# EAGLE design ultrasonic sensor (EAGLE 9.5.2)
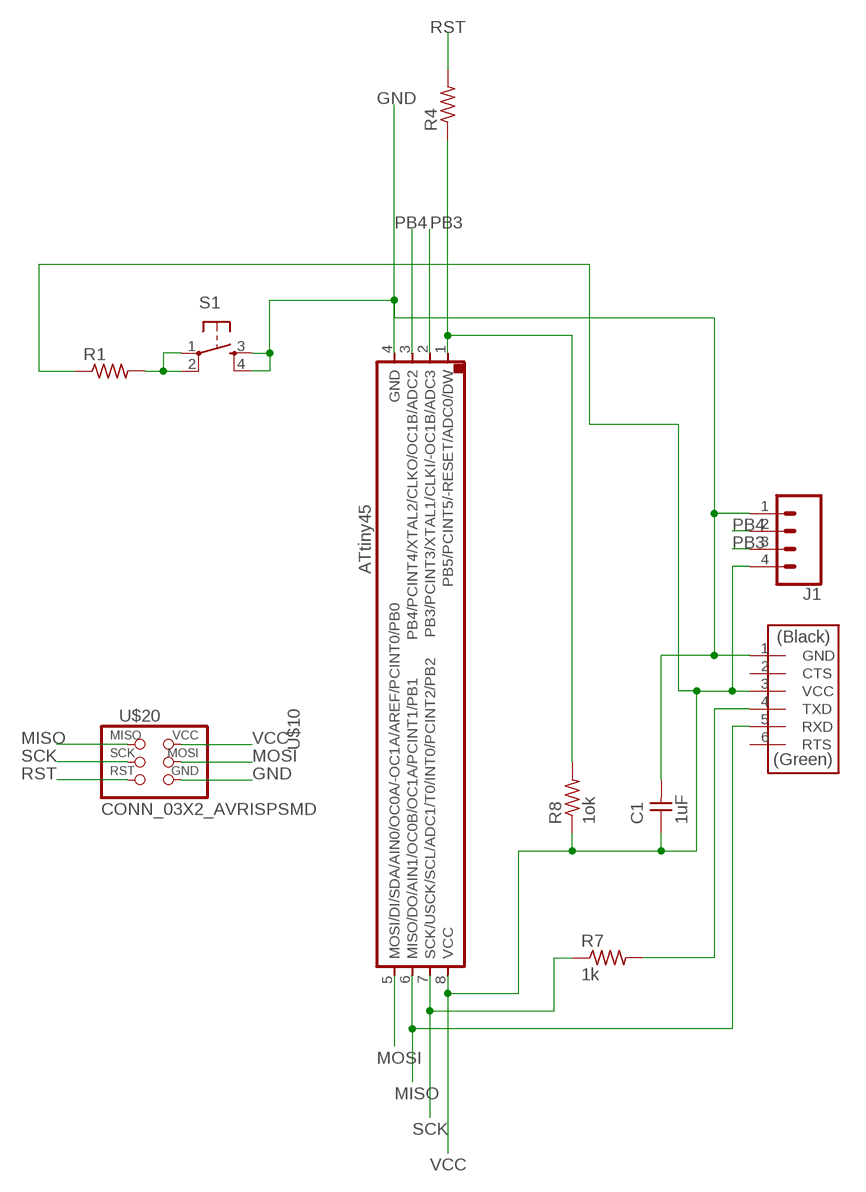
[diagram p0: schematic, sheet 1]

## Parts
C1  1uF  CAP_UNPOLARIZED  [C1206]
J1  CONN_04SMD_RA_FEMALE  [1X04_SMD_RA_FEMALE]
R1  R1206  [R1206]
R4  R1206  [R1206]
R7  1k  R1206  [R1206]
R8  1ok  R1206  [R1206]
S1  SW_SWITCH_TACTILE_6MM6MM_SWITCH  [6MM_SWITCH]
U$1  CONN_06_FTDI-SMD-HEADER  [1X06SMD]
U$10  UC_ATTINY45SI  [SOIC8]
U$20  CONN_03X2_AVRISPSMD  [2X03SMD]

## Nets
GND: C1.2 J1.1 S1.3(S) S1.4(S1) U$1.1(GND) U$10.4(GND) U$20.6(GND)
MISO: U$1.5(RXD) U$10.6(MISO/DO/AIN1/OC0B/OC1A/PCINT1/PB1) U$20.1(MISO)
MOSI: U$10.5(MOSI/DI/SDA/AIN0/OC0A/-OC1A/AREF/PCINT0/PB0) U$20.4(MOSI)
N$3: R4.1 R8.2 U$10.1(PB5/PCINT5/-RESET/ADC0/DW)
N$18: R7.2 U$1.4(TXD)
N$24: R1.2 S1.1(P) S1.2(P1)
PB3: J1.3 U$10.2(PB3/PCINT3/XTAL1/CLKI/-OC1B/ADC3)
PB4: J1.2 U$10.3(PB4/PCINT4/XTAL2/CLKO/OC1B/ADC2)
RST: R4.2 U$20.5(RST)
SCK: R7.1 U$10.7(SCK/USCK/SCL/ADC1/T0/INT0/PCINT2/PB2) U$20.3(SCK)
VCC: C1.1 J1.4 R1.1 R8.1 U$1.3(VCC) U$10.8(VCC) U$20.2(VCC)
Unconnected: U$1.2(CTS) U$1.6(RTS)

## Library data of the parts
C1 = eagle_fab:CAP_UNPOLARIZED
J1 = SparkFun-Connectors:CONN_04: Multi connection point. Often used as Generic Header-pin footprint for 0.1 inch spaced/style header connections On any of the 0.1 inch spaced packages, you can populate with these: Break Away Headers - Straight (PRT-00116) Break Away Male Headers - Right Angle (PRT-00553) Female Headers (PRT-00115)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; PROD_ID: CONN-12382
R1 R4 R7 R8 = eagle_fab:R: Resistor (US Symbol)
S1 = eagle_fab:SW_SWITCH_TACTILE_6MM: OMRON SWITCH
U$1 = eagle_fab:CONN_06_FTDI-SMD-HEADER
U$10 = eagle_fab:UC_ATTINY45
U$20 = eagle_fab:CONN_03X2_AVRISP

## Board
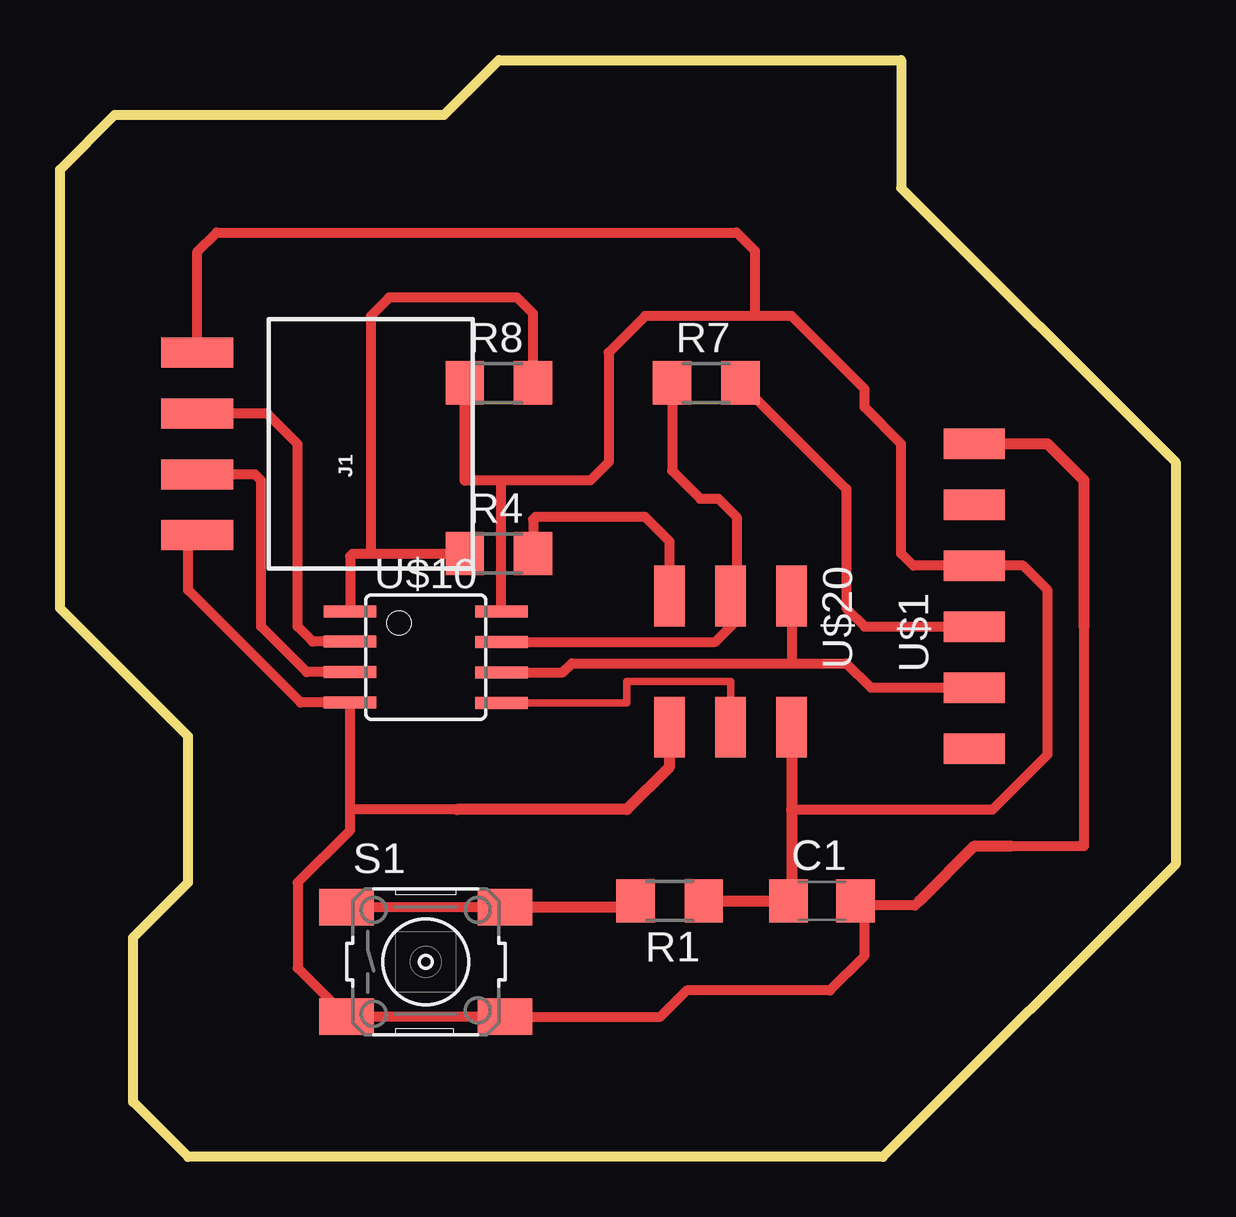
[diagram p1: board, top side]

Size 46.48 x 45.72 mm. Coordinates in mm from the lower left corner, seen from the top.
Outline: 3.05,43.43 16,43.43 18.29,45.72 35.05,45.72 35.05,40.39 46.48,28.96 46.48,12.19 34.29,0 5.33,0 3.05,2.29 3.05,9.14 5.33,11.43 5.33,17.53 0,22.86 0,41.15 2.29,43.43 4.57,43.43
Copper layers (1*16): Top 0.035mm / dielectric 1.5mm / Bottom 0.035mm
Design rules "default *": minimum track width 6mil, minimum drill 0.35mm, track to track 10mil, track to pad 6mil, pad to pad 6mil, via to via 6mil, smd to smd 6mil, copper to edge 40mil, drill to drill 6mil, minimum pad ring 10mil, minimum via ring 8mil, stop-mask expansion 4mil, vias tented up to drill 0mil, thermal gap 10mil

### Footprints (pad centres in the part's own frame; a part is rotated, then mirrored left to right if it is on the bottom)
C1206 = smd 1.6 x 1.8: 1 -1.4,0; 2 1.4,0
1X04_SMD_RA_FEMALE = smd 1.25 x 3: 1 -3.81,7.225; 2 -1.27,7.225; 3 1.27,7.225; 4 3.81,7.225
R1206 = smd 1.6 x 1.803: 1 -1.422,0; 2 1.422,0
6MM_SWITCH = smd 2.286 x 1.524: 1 -3.302,2.286; 2 3.302,2.286; 3 -3.302,-2.286; 4 3.302,-2.286
1X06SMD = smd 2.54 x 1.27: 1 0,6.35; 2 0,3.81; 3 0,1.27; 4 0,-1.27; 5 0,-3.81; 6 0,-6.35
SOIC8 = smd 0.5 x 2.2: 1 -1.905,-3.154; 2 -0.645,-3.154; 3 0.625,-3.154; 4 1.895,-3.154; 5 1.905,3.154; 6 0.635,3.154; 7 -0.635,3.154; 8 -1.905,3.154
2X03SMD = smd 2.54 x 1.27: 1 -2.54,2.54; 2 2.92,2.54; 3 -2.54,0; 4 2.92,0; 5 -2.54,-2.54; 6 2.92,-2.54

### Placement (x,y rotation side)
C1  31.75,10.67 0 top
J1  12.95,29.72 90 top
R1  25.4,10.67 180 top
R4  18.29,25.15 0 top
R7  26.92,32.26 0 top
R8  18.29,32.26 0 top
S1  15.24,8.13 0 top
U$1  38.1,23.37 0 top
U$10  15.24,20.83 270 top
U$20  27.94,20.83 270 top

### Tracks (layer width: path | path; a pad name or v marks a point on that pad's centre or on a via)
GND
  Top 0.254: 12.07,18.93 U$10.4
  Top 0.406: 39.62,12.95 42.67,12.95 42.67,22.1 | 33.34,10.48 33.53,10.29 33.53,8.38 32.08,6.93 26.11,6.93 25.02,5.84 S1.4 S1.3 9.91,7.87 9.91,11.43 12.09,13.61 12.09,14.48 | 33.34,10.48 C1.2 | 35.81,10.67 35.62,10.48 33.34,10.48 | 12.09,14.48 U$10.4 12.07,18.93 | 16.54,14.48 12.09,14.48 | U$10.4 10.02,18.93 5.33,23.62 5.33,25.51 J1.1
  Top 0.457: 16.54,14.48 23.62,14.48 25.4,16.26 U$20.6 | 39.62,12.95 38.1,12.95 35.81,10.67 | 42.67,22.1 42.67,28.19 41.15,29.72 U$1.1
MISO
  Top 0.406: U$10.6 20.96,20.19 21.34,20.57 30.48,20.57 | 30.48,20.57 32.77,20.57 33.78,19.56 U$1.5 | U$20.1 30.48,20.57
MOSI
  Top 0.305: U$20.4 27.94,19.81 23.62,19.81 23.62,18.92 U$10.5
N$3
  Top 0.406: 12.95,25.15 12.19,25.15 12.09,25.04 U$10.1 | 12.95,25.15 R4.1 | R8.2 19.71,35.15 19.05,35.81 13.72,35.81 12.95,35.05 12.95,25.15
N$18
  Top 0.406: R7.2 32.77,27.84 32.77,22.86 33.53,22.1 U$1.4
N$24
  Top 0.406: S1.1 S1.2
  Top 0.457: S1.2 23.72,10.41 R1.2
PB3
  Top 0.406: U$10.2 10.53,21.47 9.91,22.1 9.91,29.72 8.64,30.99 J1.3
PB4
  Top 0.406: U$10.3 10.28,20.2 8.38,22.1 8.38,28.19 8.13,28.45 J1.2
RST
  Top 0.406: U$20.5 25.4,25.65 24.38,26.67 19.81,26.67 19.71,26.57 R4.2
SCK
  Top 0.406: R7.1 25.5,28.6 26.67,27.43 27.43,27.43 28.19,26.67 28.19,23.62 U$20.3 28.19,23.11 28.19,22.35 27.3,21.46 U$10.7
VCC
  Top 0.254: 30.41,10.73 C1.1
  Top 0.406: 30.48,14.48 38.86,14.48 41.15,16.76 41.15,23.62 40.13,24.64 U$1.3 35.56,24.64 35.05,25.15 35.05,29.72 33.53,31.24 33.53,32 30.48,35.05 28.96,35.05 | 28.96,35.05 24.38,35.05 22.86,33.53 22.86,28.96 22.1,28.19 18.29,28.19 | 18.29,28.19 16.87,28.19 | U$10.8 18.39,28.09 18.29,28.19 | 28.96,35.05 28.96,37.77 28.19,38.53 6.53,38.53 5.73,37.73 J1.4
  Top 0.457: R1.1 C1.1 | U$20.2 30.48,14.48 30.48,10.8 30.41,10.73 | R8.1 16.87,28.19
